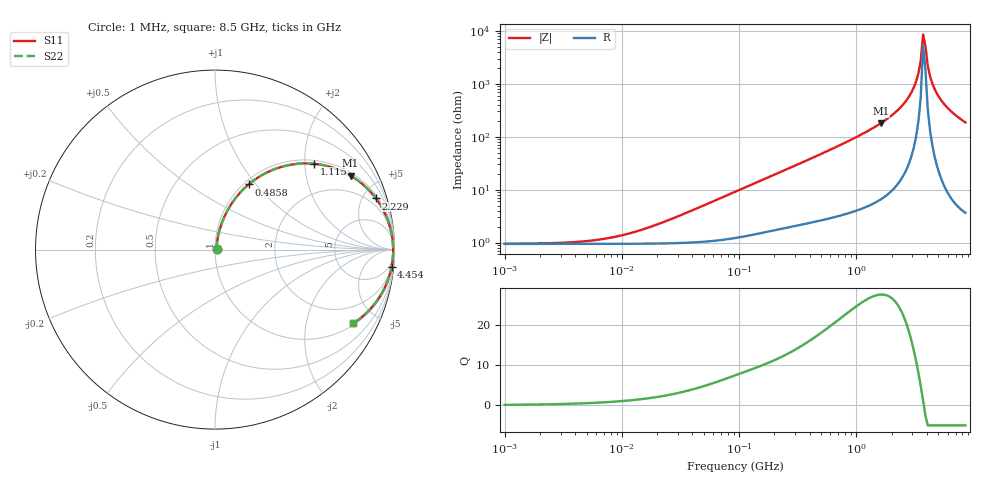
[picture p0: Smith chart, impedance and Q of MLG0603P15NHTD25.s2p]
! S-Parameter Data Generated by TDK Corporation
! Copyright(C) 2025 TDK Corporation.
! All Rights Reserved.
! TDK P/N: MLG0603P15NHTD25 (SMD / SMT Inductor (Coil))
! Property: L=15nH at 500MHz
! Size(LxWxT): 0.6x0.3x0.3mm
! Model Type: s2p (Touchstone File Format Version 1.0)
! Frequency: DC=Yes Start=1MHz Stop=8500MHz 198points Log-sweep
! Model Generated on Feb. 6, 2025
! Terms and conditions regarding TDK Simulation Models:
! 1)This simulation model is being provided solely for informational
!  purposes. Please refer to the specifications of the products in
!  terms of detailed characteristics of such products.
! 2)In no event shall TDK Corporation of any of its subsidiaries be
!  liable for any loss or damage arising, directly or indirectly,
!  from any information contained in this simulation model, including,
!  but not limited to loss or damages arising from any inaccuracies,
!  omissions or errors in connection with such information.
! 3)Any and all copyrights on this simulation model are owned by
!  TDK Corporation.  Duplication or redistribution of this simulation
!  model without prior written permission from TDK Corporation
!  is prohibited.
! 4)This simulation model is subject to any modification or change
!  without any prior notice.
! 5)Neither TDK Corporation nor any of its subsidiaries shall make any
!  warranty, express or implied, including but not limited to the
!  correctness, implied warranties of merchantability and fitness for
!  a particular purpose with respect to this simulation models.
! 6)The use of this simulation model shall be deemed to have consented
!  to the terms and conditions hereof.
! Port Assignments:
!  1 ---@@@--- 2
! Applicable Conditions:
!  Temperature = 25 degC
!  DC Bias Current = 0 A
!  Small Signal Operation
# Hz S MA R 50
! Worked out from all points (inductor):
!   197 points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, 1 MHz to 8.5 GHz, reference 50 ohm
!   read as one part in series: L = 15.7 nH near 30.45 MHz
!   highest Q = 27.5 at 1.613 GHz (marker M1), where L = 17.7 nH
!   self-resonance near 3.703 GHz
!   S11 on the Smith chart (normalised r, x): 1 MHz: 1.02, +0.00; 485.8 MHz: 1.05, +0.92; 1.115 GHz: 1.09, +2.23; 2.229 GHz: 1.25, +6.21; 4.454 GHz: 2, -20; 8.5 GHz: 1.07, -3.72
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1000000  0.009364 6.0  0.9907 -0.1  0.9907 -0.1  0.009364 6.0
4587603  0.01035 25.5  0.9907 -0.3  0.9907 -0.3  0.01035 25.5
9601846  0.01326 44.6  0.9906 -0.5  0.9906 -0.5  0.01326 44.6
2.10461e7  0.02268 64.1  0.9903 -1.2  0.9903 -1.2  0.02268 64.1
9.219544e7  0.0893 77.2  0.9841 -5.1  0.9841 -5.1  0.0893 77.2
4.229561e8  0.3631 65.3  0.9101 -21.2  0.9101 -21.2  0.3631 65.3
4.857798e8  0.4081 62.7  0.8902 -24.0  0.8902 -24.0  0.4081 62.7
1.115076e9  0.7306 40.9  0.6548 -46.9  0.6548 -46.9  0.7306 40.9
1.613203e9  0.8604 28.6  0.4793 -59.3  0.4793 -59.3  0.8604 28.6
1.940355e9  0.9109 22.3  0.3802 -65.5  0.3802 -65.5  0.9109 22.3
2.228565e9  0.9411 17.6  0.3028 -70.1  0.3028 -70.1  0.9411 17.6
2.80715e9  0.9761 9.8  0.1706 -77.1  0.1706 -77.1  0.9761 9.8
3.224109e9  0.9878 5.2  0.0903 -79.7  0.0903 -79.7  0.9878 5.2
3.37643e9  0.9902 3.6  0.0635 -79.3  0.0635 -79.3  0.9902 3.6
3.535948e9  0.9918 2.1  0.03683 -76.2  0.03683 -76.2  0.9918 2.1
3.703002e9  0.9927 0.5  0.0116 -50.8  0.0116 -50.8  0.9927 0.5
3.877948e9  0.9928 -1.0  0.0193 67.6  0.0193 67.6  0.9928 -1.0
4.061159e9  0.9921 -2.6  0.04554 78.8  0.04554 78.8  0.9921 -2.6
4.453958e9  0.9885 -5.7  0.09938 80.5  0.09938 80.5  0.9885 -5.7
4.884749e9  0.9817 -8.8  0.1534 78.8  0.1534 78.8  0.9817 -8.8
5.610304e9  0.9655 -13.5  0.2344 74.8  0.2344 74.8  0.9655 -13.5
8.5e9  0.8737 -28.0  0.4697 60.9  0.4697 60.9  0.8737 -28.0
